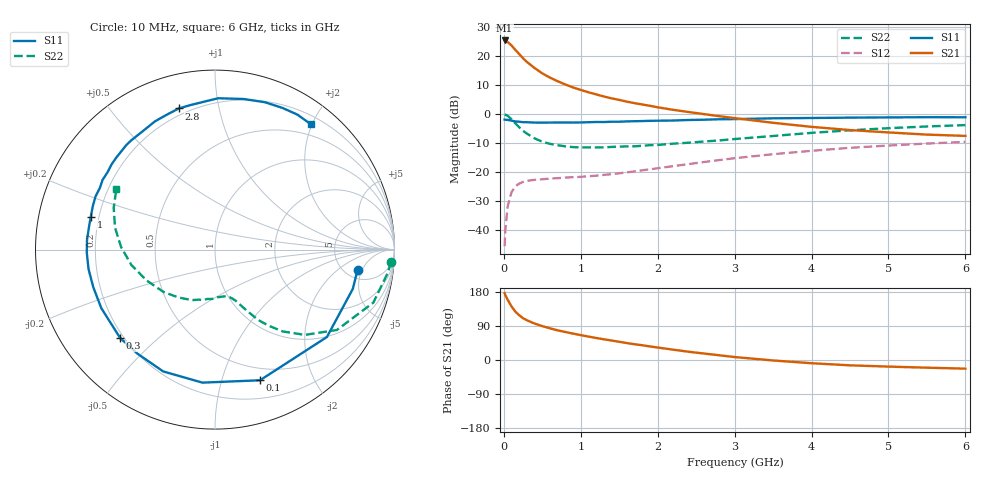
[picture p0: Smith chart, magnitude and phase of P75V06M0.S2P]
! SIEMENS Small Signal Semiconductors
! BFP196
! Si NPN RF Bipolar Junction Transistor in SOT143
! VCE = 5 V  IC = 6 mA
! Common Emitter S-Parameters:  May  1996
# GHz  S  MA  R  50
!  f  S11  S21  S12  S22
! GHz  MAG  ANG  MAG  ANG  MAG  ANG  MAG  ANG
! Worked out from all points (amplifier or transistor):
!   36 points, 10 MHz to 6 GHz, reference 50 ohm
!   highest |S21| = 25.3 dB at 10 MHz (marker M1)
!   |S21| within 3 dB of that: start of sweep to 141.2 MHz
!   unconditionally stable (mu >= 1): 1.062 GHz to 3.19 GHz
!   at 250 MHz: K = 0.29, MSG = 21.3 dB, |S12| = -23.4 dB
!   at 1.4 GHz: K = 1.14, MAG = 10.8 dB, |S12| = -20.7 dB
!   at 6 GHz: K = 0.98, MSG = 1.0 dB, |S12| = -9.6 dB
!   S11 on the Smith chart (normalised r, x): 10 MHz: 6.52, -4.09; 100 MHz: 0.37, -1.33; 300 MHz: 0.19, -0.38; 1 GHz: 0.17, +0.13; 2.8 GHz: 0.17, +0.76; 6 GHz: 0.32, +1.98
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0.01  0.8024 -8.0  18.49 176.6  0.0053 84.8  0.9831 -4.0
0.02  0.7985 -15.9  18.06 170.9  0.0104 81.1  0.9717 -7.6
0.05  0.7912 -38.0  17.39 158.9  0.0258 71.1  0.9304 -18.5
0.1  0.77 -71.0  15.19 141.4  0.0451 56.5  0.8135 -33.4
0.15  0.7445 -95.4  12.68 127.5  0.0567 45.8  0.6904 -43.5
0.2  0.7376 -113.0  10.79 118.0  0.0634 38.8  0.5904 -50.5
0.25  0.7231 -126.9  9.102 110.3  0.0677 33.8  0.5127 -55.2
0.3  0.7221 -137.1  7.876 104.8  0.0707 31.0  0.4602 -58.4
0.4  0.7125 -152.7  6.189 96.2  0.0736 27.3  0.3806 -62.7
0.5  0.7098 -162.8  5.019 89.4  0.0753 25.6  0.333 -65.8
0.6  0.7129 -171.3  4.229 83.6  0.0773 25.1  0.3065 -68.1
0.7  0.7145 -178.6  3.668 78.2  0.0786 25.1  0.2899 -70.4
0.8  0.7152 175.6  3.218 73.9  0.0803 25.8  0.2776 -72.9
1  0.7159 165.1  2.597 65.6  0.0828 28.0  0.2661 -78.0
1.1  0.7224 160.5  2.368 61.8  0.0849 29.4  0.2655 -80.8
1.6  0.7463 140.7  1.631 44.6  0.0989 35.8  0.2767 -95.5
2.2  0.7728 121.4  1.182 27.3  0.1265 40.2  0.3084 -114.1
2.8  0.8118 104.4  0.918 12.5  0.1611 39.1  0.3508 -134.2
3.5  0.8435 88.8  0.706 -1.2  0.2034 33.6  0.4185 -155.8
4.5  0.8669 71.3  0.529 -14.1  0.2618 22.7  0.524 178.3
5.5  0.8812 58.5  0.442 -20.3  0.3101 10.5  0.6104 157.6
6  0.8789 52.7  0.42 -22.8  0.3313 3.8  0.6446 148.5
